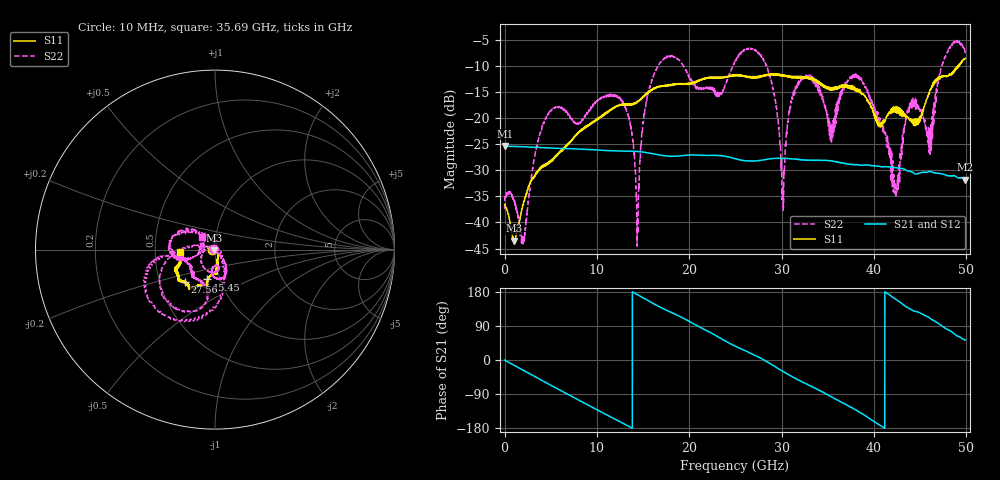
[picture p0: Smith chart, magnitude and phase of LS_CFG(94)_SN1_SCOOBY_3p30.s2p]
!Keysight Technologies,N5245B,MY58422026,A.13.80.08
!Date: Thursday, March 19, 2020 23:56:35
!Correction: S11(Full 2 Port(1,2))
!S21(Full 2 Port(1,2))
!S12(Full 2 Port(1,2))
!S22(Full 2 Port(1,2))
!S2P File: Measurements: S11, S21, S12, S22:
# Hz S DB R 50.0
!freq dBS11 angS11 dBS21 angS21 dBS12 angS12 dBS22 angS22
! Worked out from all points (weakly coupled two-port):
!   4991 points, 10 MHz to 49.91 GHz, reference 50 ohm
!   highest |S21| = -25.34 dB at 20 MHz (marker M1); lowest = -31.8 dB at 49.91 GHz (marker M2)
!   lowest |S11| = -43.5 dB at 1 GHz (marker M3), VSWR 1.01, Z = 49.5 - j0.422 ohm
!   |S11| at or under -10 dB: start of sweep to 49.12 GHz; 49.17492 GHz to 49.21963 GHz (44.71 MHz wide, 0.0909 % of centre)
!   |S22| runs from -44.6 to -5.1 dB; largest |S21 - S12| = 0.00056
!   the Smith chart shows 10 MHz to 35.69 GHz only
!   S11 on the Smith chart (normalised r, x): 10 MHz: 0.97, -0.01; 15.45 GHz: 0.87, -0.30; 27.56 GHz: 0.67, -0.26; 35.69 GHz: 0.67, -0.01
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1e7  -36.61 -169.0  -25.35 -0.3  -25.33 -0.2  -37.45 175.9
2e7  -36.56 -176.9  -25.34 -0.4  -25.35 -0.4  -35.71 -178.6
1e9  -43.52 -140.2  -25.42 -13.5  -25.42 -13.5  -35.74 -109.5
2.02e9  -36.58 -60.7  -25.48 -27.1  -25.47 -27.1  -43.26 17.0
4.44e9  -28.95 -57.1  -25.67 -59.0  -25.66 -59.0  -19.96 -141.7
8.33e9  -22.42 -79.6  -25.93 -109.8  -25.93 -109.8  -20.57 -93.4
1.267e10  -17.49 -86.8  -26.31 -164.6  -26.30 -164.5  -16.52 -66.7
1.437e10  -16.91 -98.4  -26.39 172.8  -26.37 172.9  -41.21 -99.2
1.545e10  -15.29 -104.5  -26.63 157.8  -26.62 157.8  -15.81 174.8
1.665e10  -14.02 -103.1  -27.01 141.9  -27.00 142.0  -9.91 -158.3
2.496e10  -11.84 -124.3  -27.73 36.7  -27.72 36.9  -9.24 -167.9
2.756e10  -12.09 -132.9  -28.13 7.1  -28.12 7.4  -7.73 -109.1
3.014e10  -11.85 -143.3  -27.74 -29.7  -27.75 -29.5  -33.75 29.7
3.116e10  -12.05 -146.5  -27.81 -44.1  -27.82 -43.7  -15.87 142.0
3.328e10  -12.41 -156.0  -28.06 -70.3  -28.06 -69.9  -12.21 -174.1
3.569e10  -14.19 -176.9  -28.31 -100.9  -28.25 -100.4  -19.84 135.6
3.816e10  -14.86 175.7  -28.95 -133.4  -28.89 -133.6  -11.40 -174.9
4.16e10  -18.95 108.0  -29.34 173.3  -29.37 173.2  -25.21 71.2
4.245e10  -17.99 106.6  -29.51 158.9  -29.53 158.8  -34.28 -174.7
4.39e10  -20.18 79.6  -30.20 134.8  -30.21 135.0  -17.53 -32.1
4.601e10  -15.30 8.7  -30.19 111.3  -30.22 111.5  -23.08 114.9
4.991e10  -8.54 -13.0  -31.80 52.7  -31.84 52.8  -7.32 -14.8
